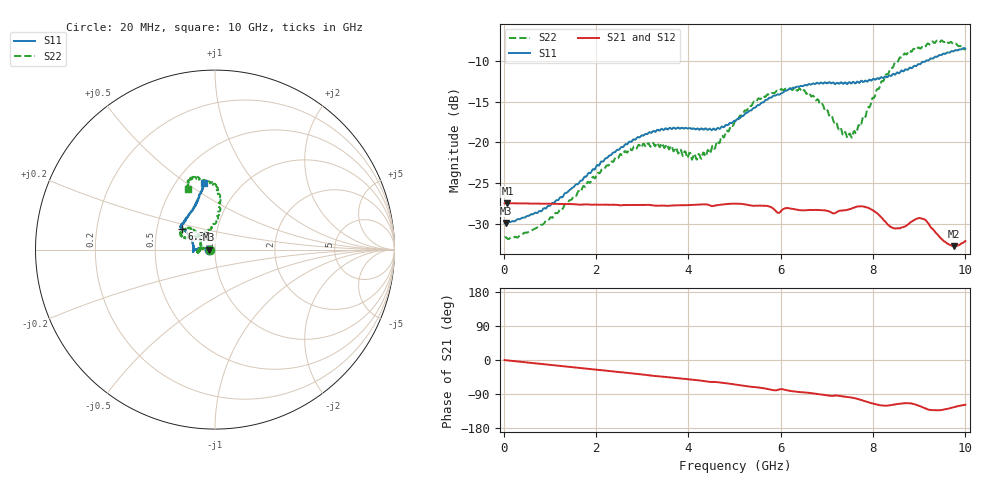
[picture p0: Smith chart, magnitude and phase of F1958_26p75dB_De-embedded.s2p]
! Integrated Device Technology
! Corporate Headquarters
! 6024 Silver Creek Valley Road
! San Jose, CA 95138  USA
! Phone:  1-408-284-8200
! Toll Free:  1-800-223-1366
! Webpage:  http://www.idt.com/
! Timing and RF Division
! 515 Groton Road, Suite 102
! Westford, MA 01886-6024
! Device:  F1958
! Description: 7-bit 0.25 dB Digital Step Attenuator
! Frequency:  0.001 -  6.000 GHz
! Package:  4x4 mm Thin QFN Plastic Package: 24 pin
! Ports:  2 RF, 12 DC
!  Pin  1  = D0
!  Pin  2  = VDD
!  Pin  3  = VMODE
!  Pin  4  = GND
!  Pin  5  = RF1  =  Port 1
!  Pin  6  = GND
!  Pin  7  = GND
!  Pin  8  = GND
!  Pin  9  = GND
!  Pin 10  = GND
!  Pin 11  = GND
!  Pin 12  = GND
!  Pin 13  = GND
!  Pin 14  = RF2  =  Port 2
!  Pin 15  = GND
!  Pin 16  = LE
!  Pin 17  = CLK
!  Pin 18  = DATA
!  Pin 19  = D6
!  Pin 20  = D5
!  Pin 21  = D4
!  Pin 22  = D3
!  Pin 23  = D2
!  Pin 24  = D1
! State:  107
! Atten State:  26.75 dB
! Voltage:  +3.30 Volts
! Current:  0.258 mA
! Data:  The device was measured on a F1958 evaluation board which has
!  individual transmission lines to the RF pins.  Data was collected
!  using a calibrated network analyzer.  The evaluation board was
!  de-embedded using Automatic Fixture Removal (AFR).
!  The reference plane is the edge of the package pin.
! Misc:
!  Action Tracker AT0419
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# GHz S dB R 50
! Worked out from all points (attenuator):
!   500 points, 20 MHz to 10 GHz, reference 50 ohm
!   highest |S21| = -27.48 dB at 80 MHz (marker M1); lowest = -32.8 dB at 9.76 GHz (marker M2)
!   lowest |S11| = -29.9 dB at 40 MHz (marker M3), VSWR 1.07, Z = 46.9 - j0.0434 ohm
!   |S11| at or under -10 dB: start of sweep to 9.139 GHz
!   |S22| runs from -31.9 to -7.5 dB; largest |S21 - S12| = 0.00033
!   S11 on the Smith chart (normalised r, x): 20 MHz: 0.94, -0.00; 6.38 GHz: 0.67, +0.16; 10 GHz: 0.68, +0.59
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0.02  -29.89 -179.0  -27.50 -0.3  -27.50 -0.3  -31.68 -178.9
0.04  -29.92 -179.2  -27.49 -0.5  -27.48 -0.5  -31.65 -178.5
0.08  -29.84 179.4  -27.48 -1.0  -27.48 -1.0  -31.84 -178.9
0.84  -28.31 171.1  -27.54 -10.9  -27.53 -10.8  -30.12 172.3
1.7  -24.68 171.0  -27.65 -21.6  -27.64 -21.6  -25.65 171.1
2.62  -20.31 176.9  -27.71 -33.2  -27.69 -33.2  -21.08 -179.9
3.36  -18.55 -176.0  -27.78 -42.9  -27.78 -43.1  -20.40 -170.0
4.24  -18.46 -179.4  -27.65 -53.9  -27.66 -54.0  -21.48 168.1
4.5  -18.51 174.7  -27.82 -58.0  -27.83 -58.0  -20.83 150.8
5.02  -17.37 160.4  -27.53 -64.8  -27.54 -64.8  -17.29 137.8
5.58  -15.13 150.2  -27.79 -73.5  -27.80 -73.6  -14.59 139.5
5.94  -14.11 148.0  -28.66 -78.9  -28.68 -78.8  -13.68 148.3
6.38  -13.16 147.9  -28.31 -84.2  -28.32 -84.2  -13.54 154.5
6.68  -12.81 146.4  -28.32 -87.7  -28.33 -87.6  -14.33 157.2
7.5  -12.64 137.9  -28.20 -98.3  -28.21 -98.2  -18.91 119.1
7.68  -12.60 135.0  -27.88 -103.1  -27.87 -103.1  -17.94 99.1
7.9  -12.41 128.6  -28.05 -111.5  -28.04 -111.5  -15.65 88.9
8.34  -11.79 118.6  -30.19 -120.0  -30.19 -120.1  -11.46 83.6
8.66  -11.29 112.8  -30.41 -114.5  -30.45 -114.4  -9.25 87.4
9.08  -10.08 106.8  -29.42 -125.0  -29.40 -125.0  -8.10 98.6
9.76  -8.75 99.8  -32.76 -124.3  -32.75 -124.1  -7.93 111.2
10  -8.46 99.6  -32.13 -118.2  -32.16 -118.5  -8.63 113.6
